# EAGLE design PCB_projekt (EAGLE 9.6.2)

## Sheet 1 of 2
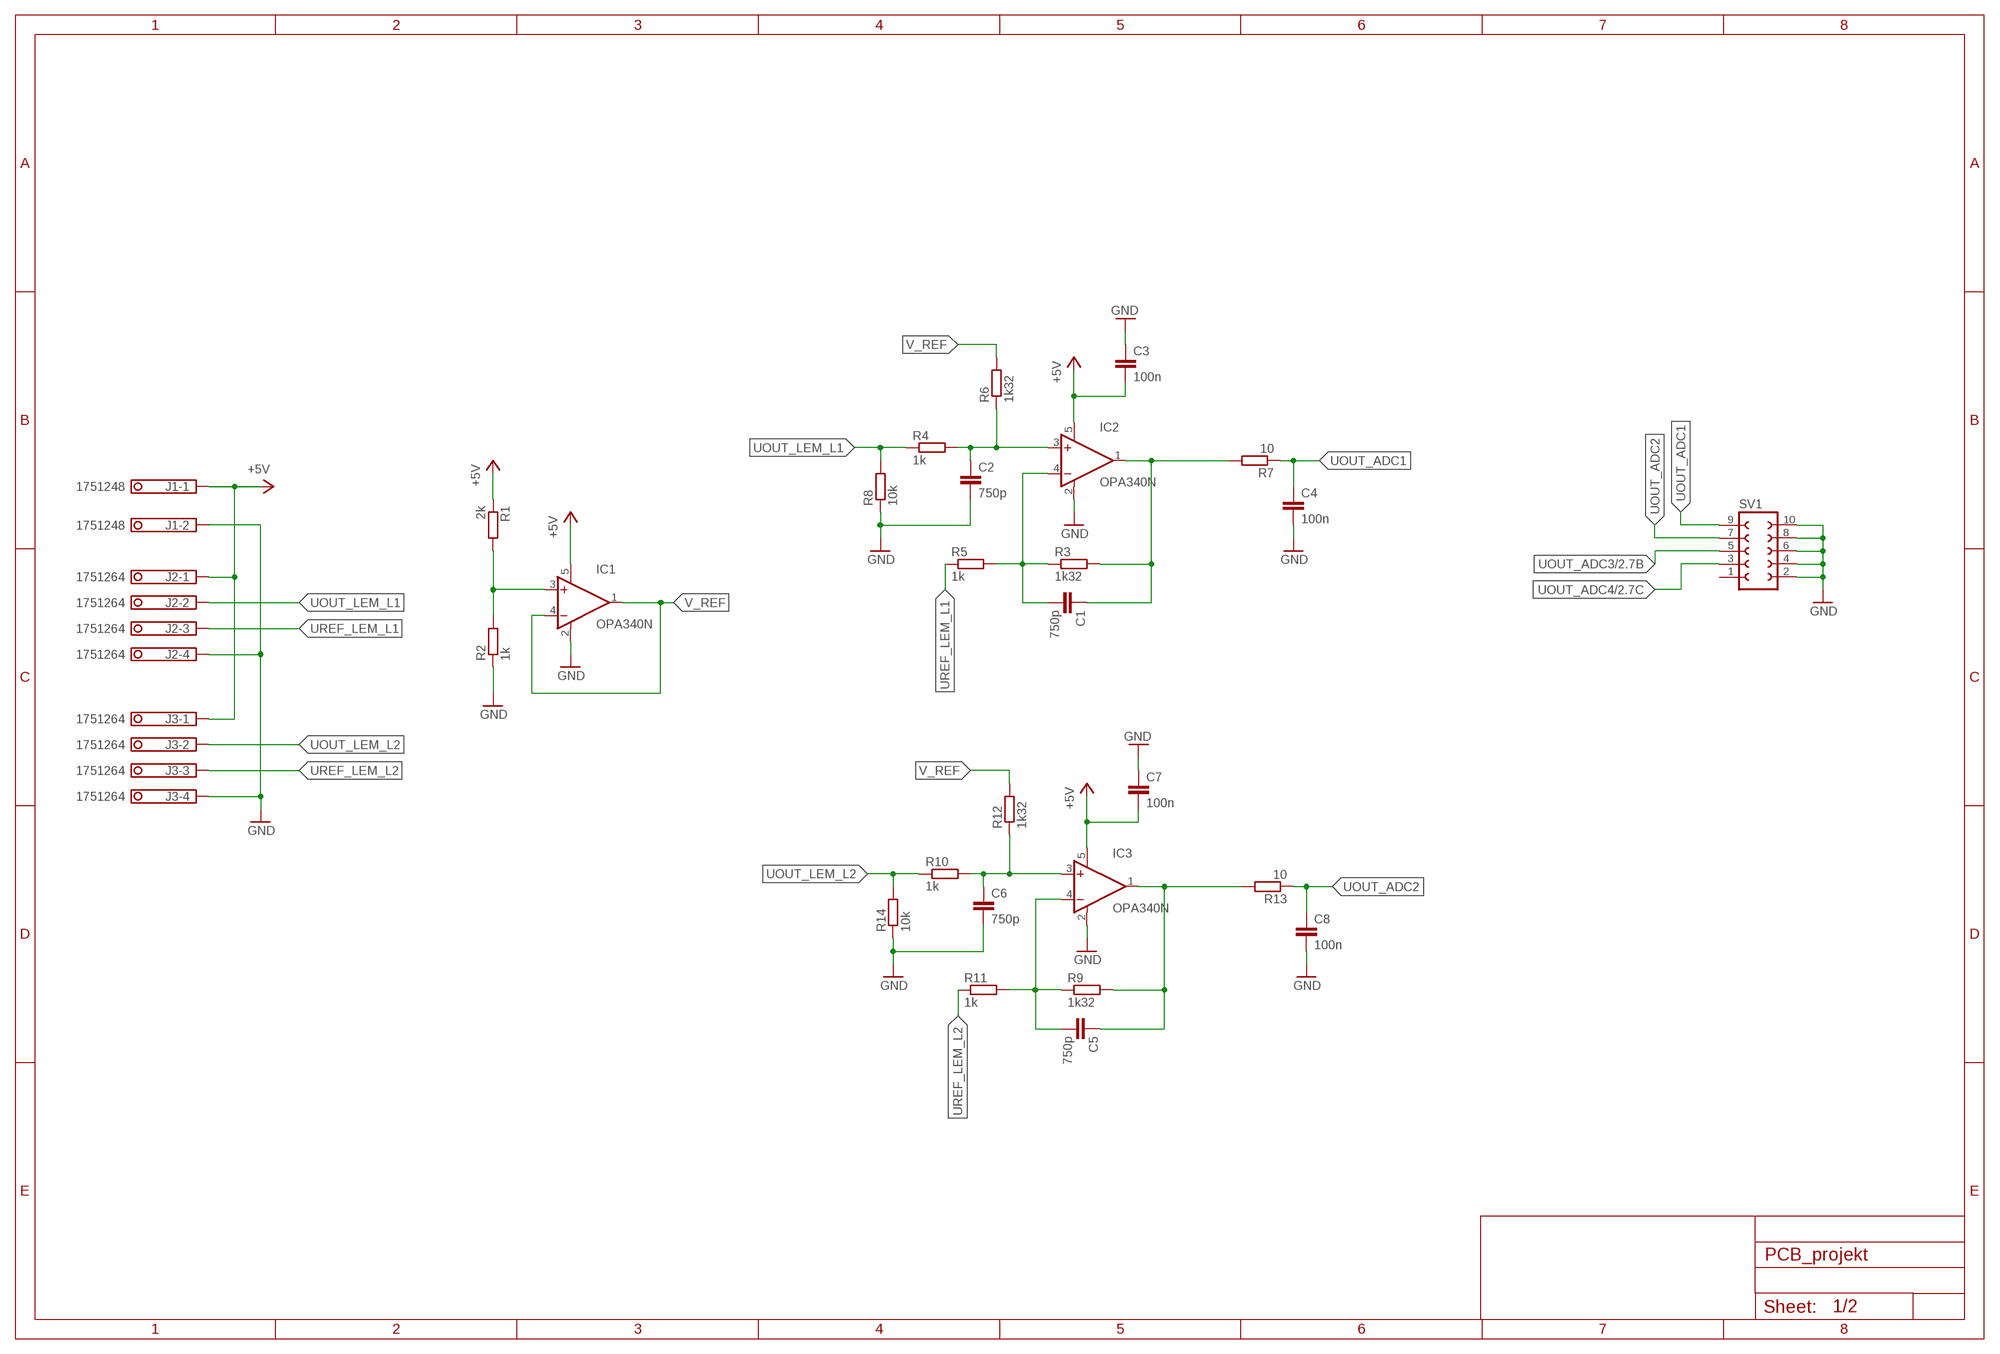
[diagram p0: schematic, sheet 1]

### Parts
C1  750p  C-EUC0603  [C0603]
C2  750p  C-EUC0603  [C0603]
C3  100n  C-EUC0603  [C0603]
C4  100n  C-EUC0603  [C0603]
C5  750p  C-EUC0603  [C0603]
C6  750p  C-EUC0603  [C0603]
C7  100n  C-EUC0603  [C0603]
C8  100n  C-EUC0603  [C0603]
IC1  OPA340N  [SOT23-5]
IC2  OPA340N  [SOT23-5]
IC3  OPA340N  [SOT23-5]
J1  1751248  [1751248]
J2  1751264  [1751264]
J3  1751264  [1751264]
R1  2k  R-EU_R1206  [R1206]
R2  1k  R-EU_R1206  [R1206]
R3  1k32  R-EU_R1206  [R1206]
R4  1k  R-EU_R1206  [R1206]
R5  1k  R-EU_R1206  [R1206]
R6  1k32  R-EU_R1206  [R1206]
R7  10  R-EU_R1206  [R1206]
R8  10k  R-EU_R1206  [R1206]
R9  1k32  R-EU_R1206  [R1206]
R10  1k  R-EU_R1206  [R1206]
R11  1k  R-EU_R1206  [R1206]
R12  1k32  R-EU_R1206  [R1206]
R13  10  R-EU_R1206  [R1206]
R14  10k  R-EU_R1206  [R1206]
SV1  FE05-2  [FE05-2]

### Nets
+5V: C3.2 C7.2 IC1.5(V+) IC2.5(V+) IC3.5(V+) J1.1 J2.1 J3.1 R1.1 ; also sheet 2
GND: C2.2 C3.1 C4.2 C6.2 C7.1 C8.2 IC1.2(V-) IC2.2(V-) IC3.2(V-) J1.2 J2.4 J3.4 R2.1 R8.1 R14.1 SV1.2 SV1.4 SV1.6 SV1.8 SV1.10 ; also sheet 2
N$1: C1.2 IC2.4(-IN) R3.1 R5.2
N$2: C1.1 IC2.1(OUT) R3.2 R7.2
N$4: IC1.3(+IN) R1.2 R2.2
N$5: C2.1 IC2.3(+IN) R4.2 R6.1
N$9: C5.2 IC3.4(-IN) R9.1 R11.2
N$10: C5.1 IC3.1(OUT) R9.2 R13.2
N$11: C6.1 IC3.3(+IN) R10.2 R12.1
UOUT_ADC1: C4.1 R7.1 SV1.9
UOUT_ADC2: C8.1 R13.1 SV1.7
UOUT_ADC3: SV1.5 ; also sheet 2
UOUT_ADC4: SV1.3 ; also sheet 2
UOUT_LEM_L1: J2.2 R4.1 R8.2
UOUT_LEM_L2: J3.2 R10.1 R14.2
UREF_LEM_L1: J2.3 R5.1
UREF_LEM_L2: J3.3 R11.1
V_REF: IC1.1(OUT) IC1.4(-IN) R6.2 R12.2
Unconnected: SV1.1

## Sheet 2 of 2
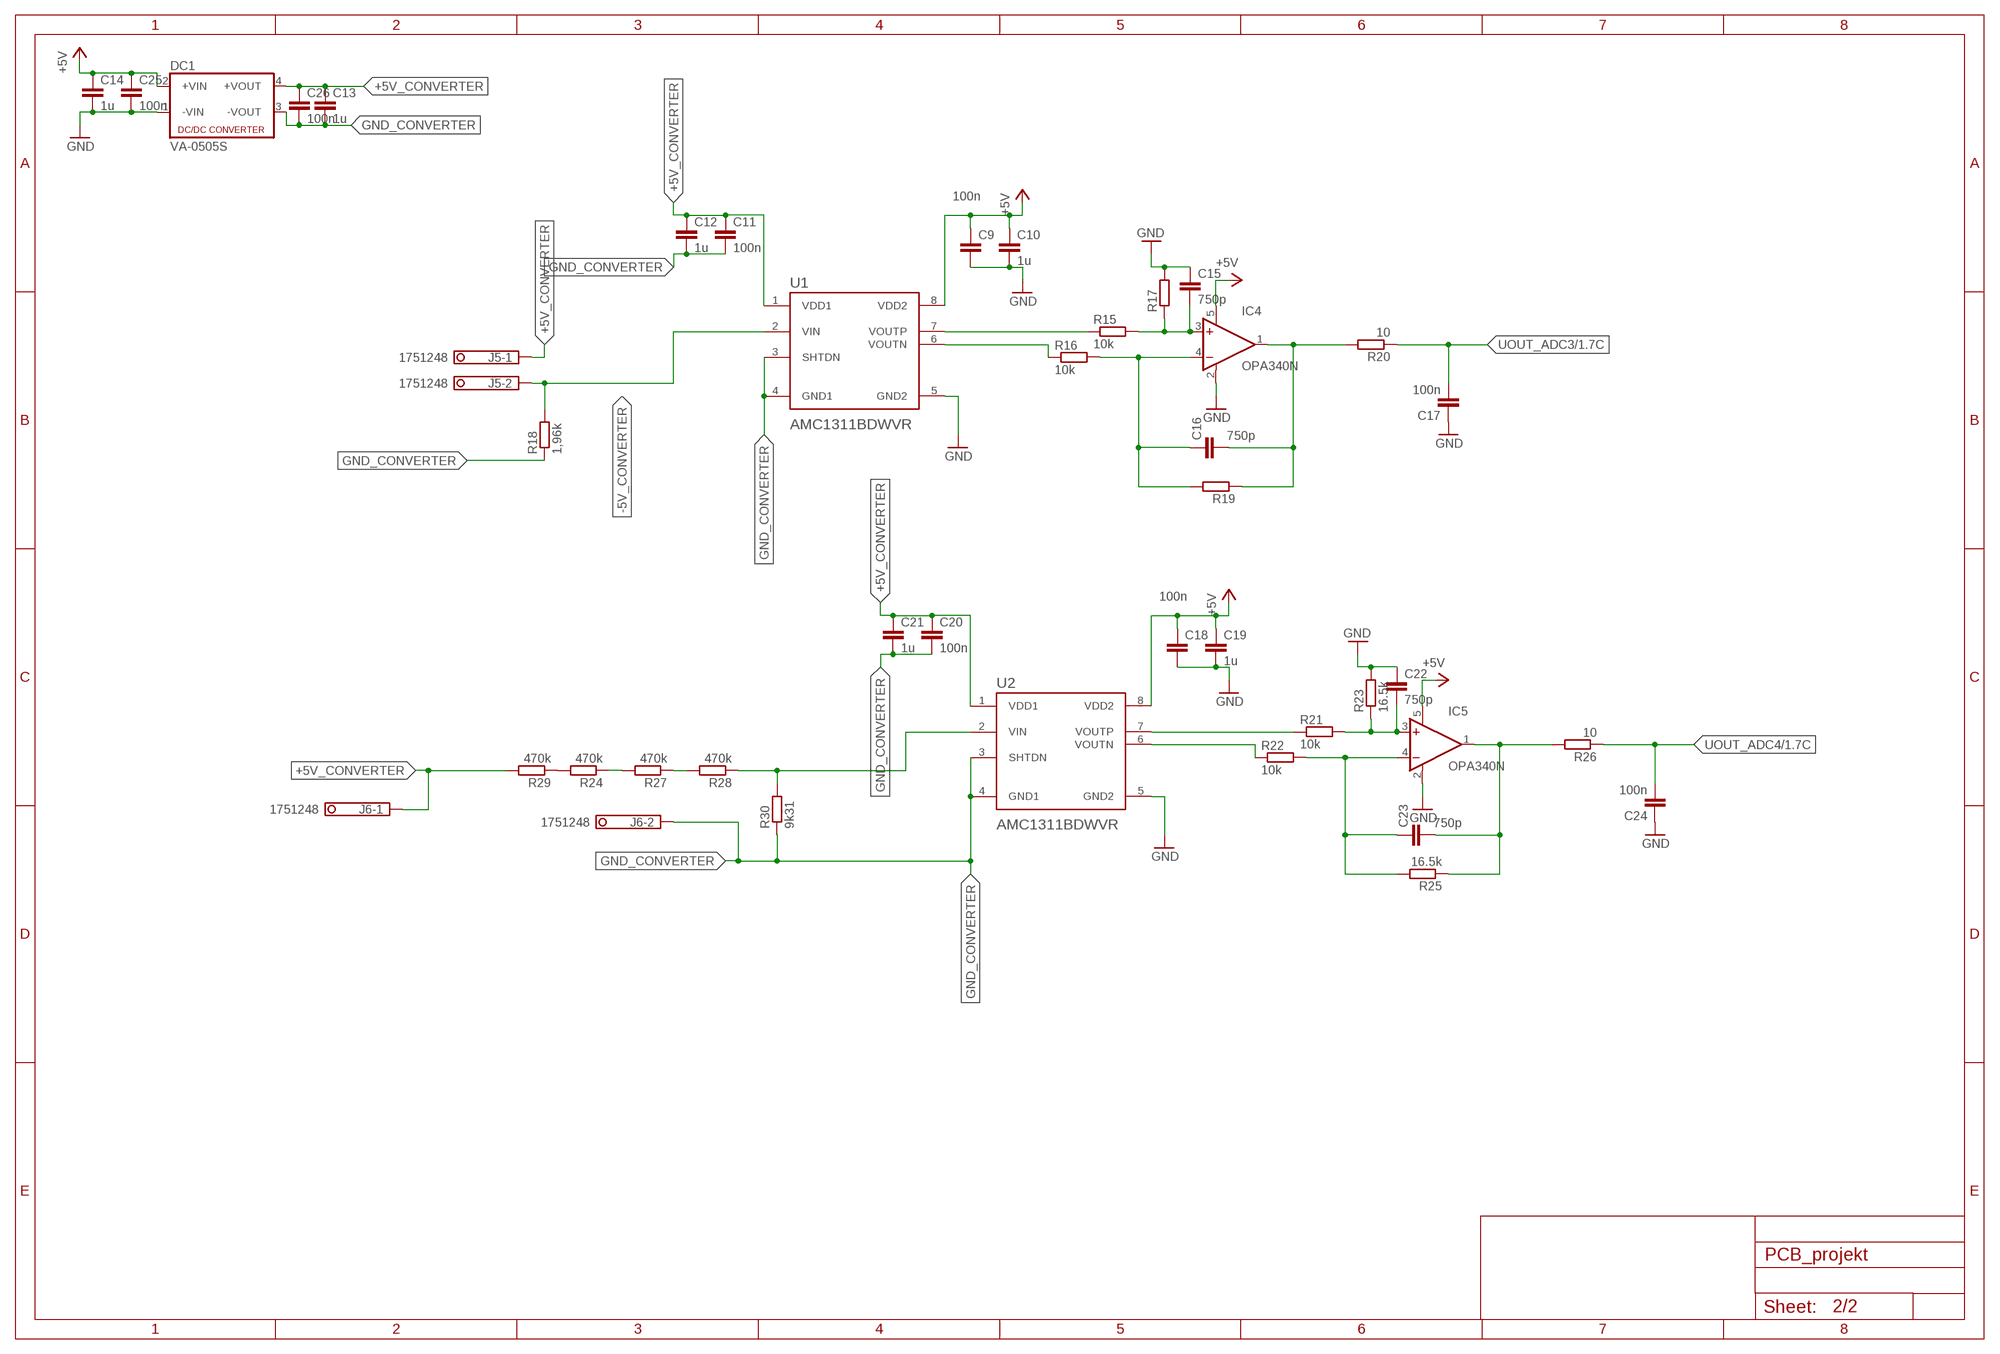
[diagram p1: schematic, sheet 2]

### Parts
C9  100n  C-EUC0603  [C0603]
C10  1u  C-EUC0603  [C0603]
C11  100n  C-EUC0603  [C0603]
C12  1u  C-EUC0603  [C0603]
C13  1u  C-EUC0603  [C0603]
C14  1u  C-EUC0603  [C0603]
C15  750p  C-EUC0603  [C0603]
C16  750p  C-EUC0603  [C0603]
C17  100n  C-EUC0603  [C0603]
C18  100n  C-EUC0603  [C0603]
C19  1u  C-EUC0603  [C0603]
C20  100n  C-EUC0603  [C0603]
C21  1u  C-EUC0603  [C0603]
C22  750p  C-EUC0603  [C0603]
C23  750p  C-EUC0603  [C0603]
C24  100n  C-EUC0603  [C0603]
C25  100n  C-EUC0603  [C0603]
C26  100n  C-EUC0603  [C0603]
DC1  VA-0505S  [4SIL]
IC4  OPA340N  [SOT23-5]
IC5  OPA340N  [SOT23-5]
J5  1751248  [1751248]
J6  1751248  [1751248]
R15  10k  R-EU_R1206  [R1206]
R16  10k  R-EU_R1206  [R1206]
R17  R-EU_R1206  [R1206]
R18  1,96k  R-EU_R1206  [R1206]
R19  R-EU_R1206  [R1206]
R20  10  R-EU_R1206  [R1206]
R21  10k  R-EU_R1206  [R1206]
R22  10k  R-EU_R1206  [R1206]
R23  16.5k  R-EU_R1206  [R1206]
R24  470k  R-EU_R1206  [R1206]
R25  16.5k  R-EU_R1206  [R1206]
R26  10  R-EU_R1206  [R1206]
R27  470k  R-EU_R1206  [R1206]
R28  470k  R-EU_R1206  [R1206]
R29  470k  R-EU_R1206  [R1206]
R30  9k31  R-EU_R1206  [R1206]
U1  AMC1311BDWVR  [SOIC127P1150X280-8N]
U2  AMC1311BDWVR  [SOIC127P1150X280-8N]

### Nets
+5V: C9.1 C10.1 C14.1 C18.1 C19.1 C25.1 DC1.2(+VIN) IC4.5(V+) IC5.5(V+) U1.8(VDD2) U2.8(VDD2) ; also sheet 1
+5V_CONVERTER: C11.1 C12.1 C13.1 C20.1 C21.1 C26.1 DC1.4(+VOUT) J5.1 J6.1 R29.2 U1.1(VDD1) U2.1(VDD1)
-5V_CONVERTER: J5.2 R18.2 U1.2(VIN)
GND: C9.2 C10.2 C14.2 C15.1 C17.1 C18.2 C19.2 C22.1 C24.1 C25.2 DC1.1(-VIN) IC4.2(V-) IC5.2(V-) R17.2 R23.2 U1.5(GND2) U2.5(GND2) ; also sheet 1
GND_CONVERTER: C11.2 C12.2 C13.2 C20.2 C21.2 C26.2 DC1.3(-VOUT) J6.2 R18.1 R30.1 U1.3(SHTDN) U1.4(GND1) U2.3(SHTDN) U2.4(GND1)
N$15: R15.1 U1.7(VOUTP)
N$16: R16.1 U1.6(VOUTN)
N$17: C16.2 IC4.1(OUT) R19.1 R20.2
N$18: C16.1 IC4.4(-IN) R16.2 R19.2
N$19: C15.2 IC4.3(+IN) R15.2 R17.1
N$22: R24.2 R29.1
N$25: R21.1 U2.7(VOUTP)
N$26: R22.1 U2.6(VOUTN)
N$27: C23.2 IC5.1(OUT) R25.1 R26.2
N$28: C23.1 IC5.4(-IN) R22.2 R25.2
N$29: C22.2 IC5.3(+IN) R21.2 R23.1
N$33: R24.1 R27.2
N$34: R27.1 R28.2
N$35: R28.1 R30.2 U2.2(VIN)
UOUT_ADC3: C17.2 R20.1 ; also sheet 1
UOUT_ADC4: C24.2 R26.1 ; also sheet 1

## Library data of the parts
C1-C26 = rcl:C-EU: CAPACITOR, European symbol; SPICEPREFIX: C
DC1 = dc-dc-converter:VA-*?: DC DC Converter Single Output, 1 Watt Motien Technology Co.,Ltd. Source: Data sheet; OC_FARNELL: unknown; OC_NEWARK: unknown
IC1-IC5 = burr-brown:OPA340: Rail-to-Rail Operational Amplifiers Single-Supply, MicroAmplifier(TM) Series; MPN: OPA340NA/3KG4; OC_FARNELL: 1234805; OC_NEWARK: 13M5177
J1 J5 J6 = con-phoenix-350:1751248: MKDS 1/ 2-3,5 Printklemme; OC_FARNELL: unknown; OC_NEWARK: unknown
J2 J3 = con-phoenix-350:1751264: MKDS 1/ 4-3,5 Printklemme Nennstrom: 10 A Bemessungsspannung: 160 V Raster: 3,5 mm Polzahl: 4 Montageart: Löten Anschlussart: Schraubanschluss Anschlussrichtung vom Leiter zur Platine: 0° Source: http://eshop.phoenixcontact.com .. 1751264.pdf; MPN: 1751264; OC_FARNELL: unknown; OC_NEWARK: 10R0934
R1-R30 = rcl:R-EU_: RESISTOR, European symbol; SPICEPREFIX: R
SV1 = con-lsta:FE05-2: FEMALE HEADER; OC_FARNELL: unknown; OC_NEWARK: unknown
U1 U2 = AMC1311BDWVR:AMC1311BDWVR: Check availability; AVAILABILITY: In Stock; CHECK_PRICES: https://www.snapeda.com/parts/AMC1311BDWVR/Texas+Instruments/view-part/?ref=eda; DESCRIPTION: 2-V input, precision voltage sensing reinforced isolated amplifier; MF: Texas Instruments; MP: AMC1311BDWVR; PACKAGE: SOIC-8 Texas Instruments; PRICE: None; PURCHASE-URL: https://www.snapeda.com/api/url_track_click_mouser/?unipart_id=3594462&manufacturer=Texas Instruments&part_name=AMC1311BDWVR&search_term=None; SNAPEDA_LINK: https://www.snapeda.com/parts/AMC1311BDWVR/Texas+Instruments/view-part/?ref=snap

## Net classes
0 default: width 0.3 mm, drill 0.3 mm

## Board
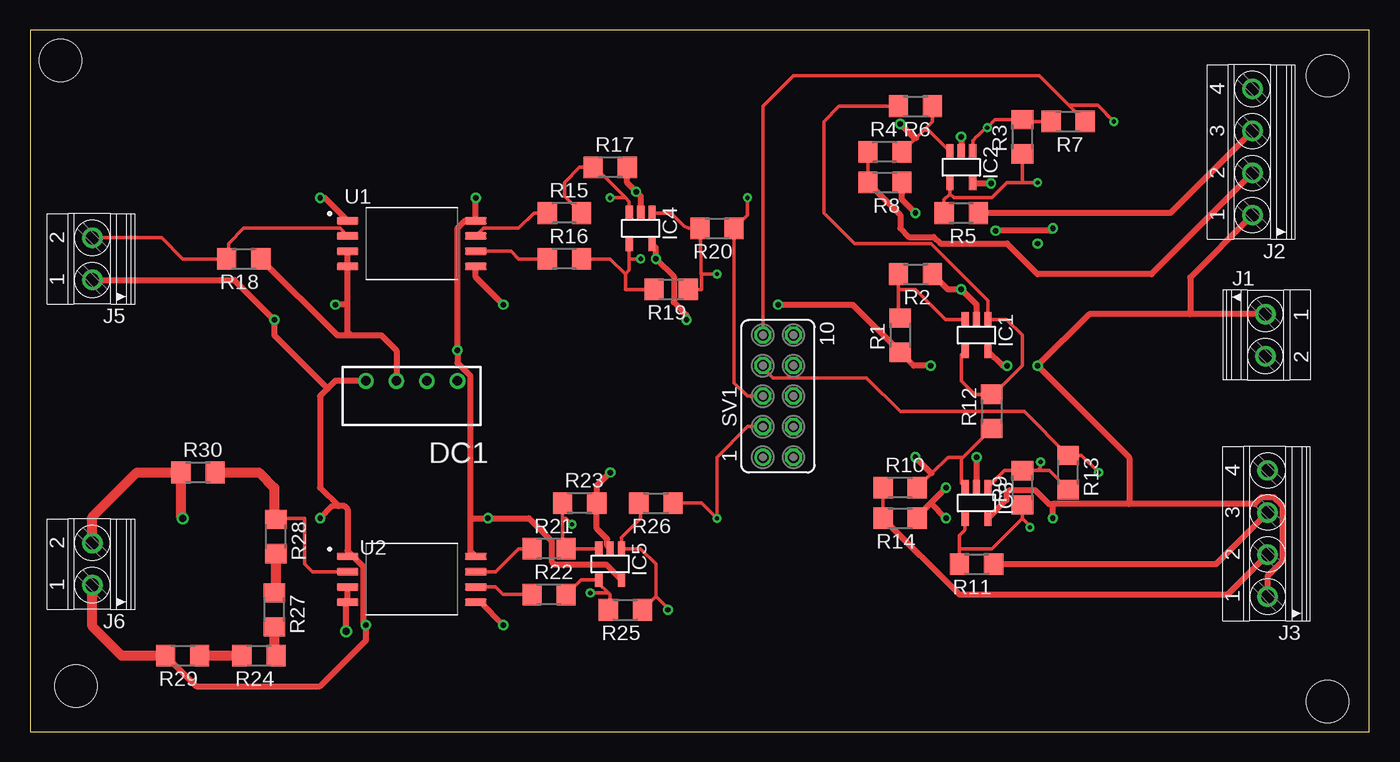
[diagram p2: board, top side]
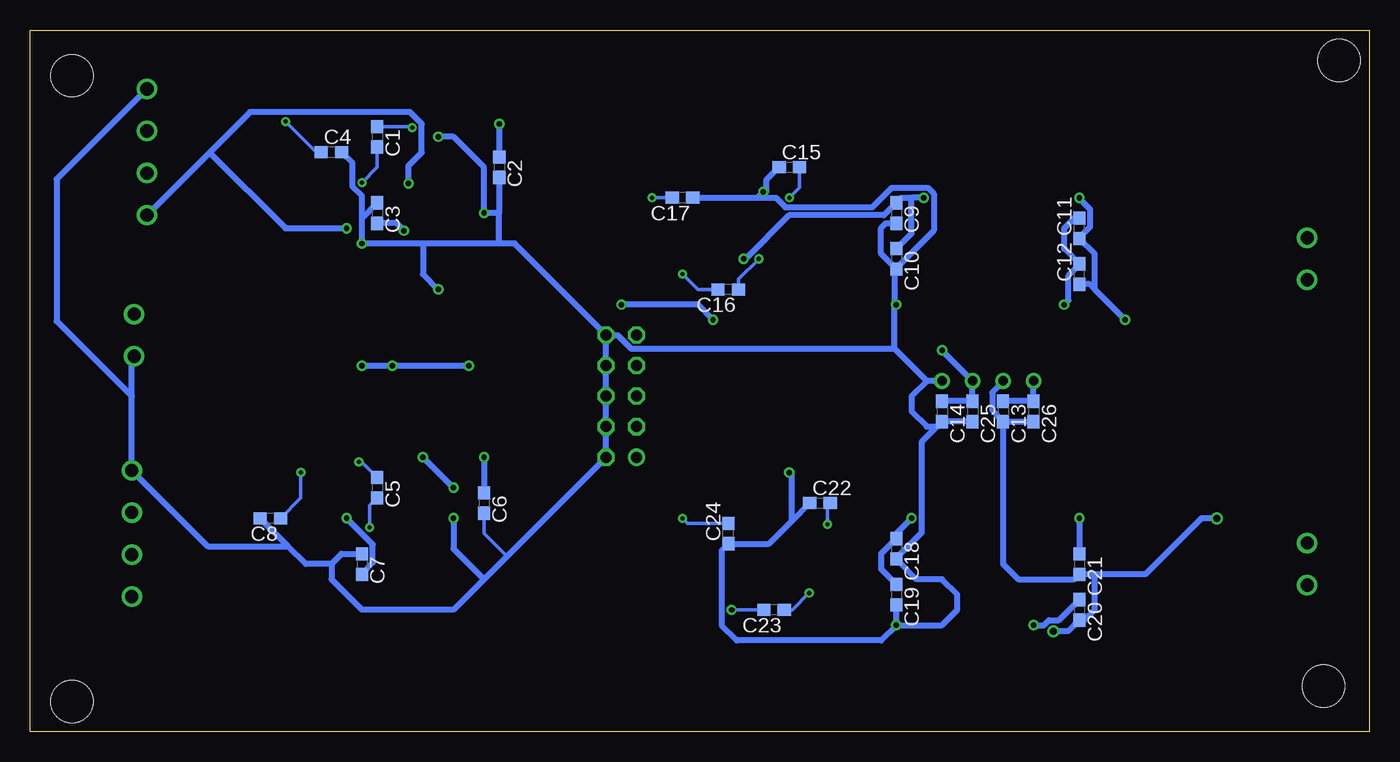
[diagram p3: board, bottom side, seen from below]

Size 111.43 x 58.41 mm. Coordinates in mm from the lower left corner, seen from the top.
Outline: 0,0 111.43,0 111.43,58.41 0,58.41 0,0
Copper layers (1*16): Top 0.035mm / dielectric 1.5mm / Bottom 0.035mm
Design rules "default": minimum track width 6mil, minimum drill 0.35mm, track to track 6mil, track to pad 6mil, pad to pad 6mil, via to via 6mil, smd to smd 6mil, copper to edge 40mil, drill to drill 6mil, minimum pad ring 10mil, minimum via ring 8mil, stop-mask expansion 4mil, vias tented up to drill 0mil, thermal gap 10mil
Holes 3.5 mm at 2.54,55.88 3.81,3.81 107.95,2.54 107.95,54.61

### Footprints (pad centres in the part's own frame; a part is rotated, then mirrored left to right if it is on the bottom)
C0603 = smd 1.1 x 1: 1 -0.85,0; 2 0.85,0
4SIL = drill 0.8: 1 -3.81,0; 2 -1.27,0; 3 1.27,0; 4 3.81,0
SOT23-5 = smd 0.6 x 1.2: 1 -0.95,-1.306; 2 0,-1.306; 3 0.95,-1.306; 4 0.95,1.306; 5 -0.95,1.306
1751248 = drill 1.1 pad 1.7: 1 -1.75,-0.1; 2 1.75,-0.1
1751264 = drill 1.1 pad 1.7: 1 -5.25,-0.1; 2 -1.75,-0.1; 3 1.75,-0.1; 4 5.25,-0.1
R1206 = smd 1.6 x 1.803: 1 -1.422,0; 2 1.422,0
FE05-2 = drill 0.914: 1 -5.08,1.27 | drill 0.914 octagon: 2 -5.08,-1.27; 3 -2.54,1.27; 4 -2.54,-1.27; 5 0,1.27; 6 0,-1.27; 7 2.54,1.27; 8 2.54,-1.27; 9 5.08,1.27; 10 5.08,-1.27
SOIC127P1150X280-8N = smd 1.8 x 0.6: 1 -5.33,1.905; 2 -5.33,0.635; 3 -5.33,-0.635; 4 -5.33,-1.905; 5 5.33,-1.905; 6 5.33,-0.635; 7 5.33,0.635; 8 5.33,1.905

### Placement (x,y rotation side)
C1  82.55,49.53 270 bottom
C2  72.39,46.99 270 bottom
C3  82.55,43.18 270 bottom
C4  86.36,48.26 0 bottom
C5  82.55,20.32 270 bottom
C6  73.66,19.05 270 bottom
C7  83.82,13.97 270 bottom
C8  91.44,17.78 180 bottom
C9  39.37,43.18 270 bottom
C10  39.37,39.37 270 bottom
C11  24.13,41.91 90 bottom
C12  24.13,38.1 90 bottom
C13  30.48,26.67 270 bottom
C14  35.56,26.67 270 bottom
C15  48.26,46.99 0 bottom
C16  53.34,36.83 180 bottom
C17  57.15,44.45 180 bottom
C18  39.37,15.24 270 bottom
C19  39.37,11.43 270 bottom
C20  24.13,10.16 270 bottom
C21  24.13,13.97 270 bottom
C22  45.72,19.05 0 bottom
C23  49.53,10.16 180 bottom
C24  53.34,16.51 90 bottom
C25  33.02,26.67 270 bottom
C26  27.94,26.67 270 bottom
DC1  31.75,29.21 180 top
IC1  78.74,33.02 180 top
IC2  77.47,46.99 180 top
IC3  78.74,19.05 180 top
IC4  50.8,41.91 180 top
IC5  48.26,13.97 180 top
J1  102.87,33.02 270 top
J2  101.6,48.26 90 top
J3  102.87,16.51 90 top
J5  5.08,39.37 90 top
J6  5.08,13.97 90 top
R1  72.39,33.02 90 top
R2  73.66,38.1 180 top
R3  82.55,49.53 90 top
R4  71.12,48.26 0 top
R5  77.47,43.18 180 top
R6  73.66,52.07 180 top
R7  86.36,50.8 180 top
R8  71.12,45.72 180 top
R9  82.55,20.32 90 top
R10  72.39,20.32 0 top
R11  78.74,13.97 180 top
R12  80.01,26.67 90 top
R13  86.36,21.59 270 top
R14  72.39,17.78 180 top
R15  44.45,43.18 0 top
R16  44.45,39.37 0 top
R17  48.26,46.99 0 top
R18  17.78,39.37 180 top
R19  53.34,36.83 180 top
R20  57.15,41.91 180 top
R21  43.18,15.24 0 top
R22  43.18,11.43 0 top
R23  45.72,19.05 0 top
R24  19.05,6.35 180 top
R25  49.53,10.16 180 top
R26  52.07,19.05 180 top
R27  20.32,10.16 270 top
R28  20.45,16.26 270 top
R29  12.7,6.35 180 top
R30  13.97,21.59 0 top
SV1  62.23,27.94 90 top
U1  31.75,40.64 0 top
U2  31.75,12.7 0 top

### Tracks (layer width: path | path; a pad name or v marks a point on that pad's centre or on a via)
+5V  (via drill 0.45)
  Top 0.508: U2.8 36.62,15.07 36.62,17.78 | 36.62,17.78 36.62,29.65 35.56,30.71 v35.56,31.75 35.56,41.91 36.2,42.55 U1.8 v37.08,44.45 | 36.62,17.78 v38.1,17.78 41.49,17.78 43.4,15.88 43.4,14.17 43.63,13.93 47.94,13.93 IC5.5 | IC4.5 52.07,40.28 v52.07,39.37 53.56,37.88 53.56,35.76 54.61,34.71 v54.61,34.29 | v62.23,35.56 68.43,35.56 R1.1 73.51,30.48 v74.93,30.48 | J3.1 102.97,12.98 104.05,14.06 104.23,14.24 104.23,18.78 104.05,18.96 103.49,19.52 102.45,19.52 101.89,18.96 91.44,18.96 | IC3.5 81.24,19.3 81.24,19.87 81.48,20.1 83.62,20.1 84.76,18.96 85.09,18.96 | 91.44,18.96 85.09,18.96 | v85.09,17.78 85.09,18.96 | J1.1 96.52,34.77 | 96.52,34.77 88.11,34.77 v83.82,30.48 91.44,22.86 91.44,18.96 | v81.28,30.48 80.92,30.48 IC1.5 | IC2.5 79.91,45.68 v79.94,45.65 | v85.09,41.91 84.9,41.72 v80.33,41.72 | J2.1 96.52,37.83 96.52,34.77
  Bottom 0.508: C14.1 C25.1 DC1.2 v35.56,31.75 | v38.1,17.78 39.37,16.51 C18.1 40.64,14.82 40.64,13.55 C19.1 | 38.1,44.45 38.95,44.45 C9.1 40.41,42.99 48.29,42.99 51.91,39.37 v52.07,39.37 | v37.08,44.45 38.1,44.45 | C10.1 38.1,41.49 38.1,44.45 | v54.61,34.29 55.88,35.56 v62.23,35.56 | C7.2 83.82,13.19 82.91,14.1 82.91,15.6 v85.09,17.78 | v83.82,30.48 v81.28,30.48 v74.93,30.48 | 96.48,48.22 93.12,51.58 79.81,51.58 78.84,50.62 78.84,48.22 79.94,47.12 v79.94,45.65 | 96.48,48.22 J2.1 | 96.48,48.22 90.17,41.91 v85.09,41.91 | v80.33,41.72 80.95,42.33 C3.2
+5V_CONVERTER  (via drill 0.45)
  Top 0.508: DC1.4 25.4,29.21 24.77,28.57 | 24.77,28.57 24.13,27.94 24.13,20.32 25.65,18.8 | 25.65,18.8 26.16,18.8 26.42,18.54 26.42,15.07 | 26.42,15.07 U2.1 | 25.65,18.8 25.15,18.8 v24.13,17.78 | 24.77,28.57 20.32,33.02 v20.32,34.29 16.99,37.62 J5.1 | v24.13,44.45 24.52,44.45 U1.1 | 26.42,15.07 27.73,13.76 27.73,9.1 v27.94,8.89 27.94,7.62 24.13,3.81 13.82,3.81 R29.2
  Top 0.813: R29.2 7.62,6.35 5.18,8.79 J6.1
  Bottom 0.508: v24.13,17.78 C21.1 | DC1.4 C26.1 C13.1 | v20.32,34.29 22.86,36.83 | 22.86,36.83 23.28,37.25 C12.1 | 22.86,36.83 22.86,39.79 C11.1 24.13,41.14 23.22,42.04 23.22,43.48 24.13,44.38 v24.13,44.45 | v27.94,8.89 27.07,8.89 26.67,9.29 25.85,9.29 C20.1
-5V_CONVERTER
  Top 0.3: J5.2 10.95,41.12 12.7,39.37 R18.2 16.43,39.45 16.51,39.52 16.51,40.64 17.78,41.91 25.79,41.91 U1.2
GND  (via drill 0.45)
  Top 0.508: v39.37,8.89 37.47,10.79 U2.5 | IC5.2 48.02,15.52 48.02,16.04 47.14,16.92 R23.2 47.14,20.47 v48.26,21.59 | v39.37,35.56 37.08,37.85 U1.5 | IC4.2 50.8,44.58 v50.42,44.96 49.68,45.69 R17.2 | v78.74,22.86 IC3.2 | R2.1 76.35,36.83 v77.47,36.83 78.74,35.56 IC1.2 | v73.66,43.18 72.54,44.3 R8.1 | v77.47,49.53 IC2.2 | 74.93,19.05 73.81,17.93 R14.1 | 74.93,19.05 v76.2,17.78 | 74.93,19.05 v76.2,20.32
  Bottom 0.3: C6.2 73.45,17.99 73.66,17.78 73.66,16.51 71.75,14.61
  Bottom 0.508: DC1.1 36.83,29.21 | 36.83,29.21 38.1,27.94 38.1,26.67 36.83,25.4 35.98,25.4 C14.2 | C25.2 C14.2 | 39.16,14.18 C18.2 39.16,14.6 | 39.16,14.18 37.68,12.7 35.56,12.7 34.29,11.43 34.29,10.16 35.56,8.89 v39.37,8.89 | v39.37,8.89 C19.2 | 48.05,17.57 49.96,15.66 C24.1 53.9,15.1 53.9,8.89 52.63,7.62 40.64,7.62 v39.37,8.89 | 48.05,17.57 C22.1 | SV1.10 SV1.8 SV1.6 SV1.4 SV1.2 71.75,14.61 73.66,12.7 | SV1.10 62.54,33.02 61.42,31.9 39.52,31.9 | 36.83,29.21 39.52,31.9 | 39.52,31.9 39.52,35.41 | 39.52,35.41 v39.37,35.56 | C10.2 39.52,38.37 39.52,35.41 | C10.2 40.64,39.79 40.64,41.91 40.22,42.33 C9.2 | C17.1 50.93,44.45 | 50.93,44.45 v50.42,44.96 50.19,44.96 50.19,45.91 C15.1 | 50.93,44.45 49.37,44.45 48.59,43.66 41.36,43.66 39.74,45.28 36.73,45.28 36.24,44.8 36.24,41.72 39.37,38.59 C10.2 | SV1.10 71.12,40.64 72.39,40.64 | 72.39,40.64 78.74,40.64 | 78.74,40.64 v83.82,40.64 83.82,42.76 | 83.82,42.76 C3.1 | 83.82,42.76 83.82,44.61 84.61,45.39 84.61,47.35 C4.2 | 72.39,40.64 72.39,43.18 | C2.2 72.39,43.18 | 73.66,12.7 76.2,10.16 83.82,10.16 86.36,12.7 86.36,13.97 | 86.36,13.97 85.51,14.82 C7.1 | 86.36,13.97 88.48,13.97 89.96,15.45 | 89.96,15.45 C8.2 | 89.96,15.45 96.66,15.45 J3.4 102.97,27.94 | 102.97,27.94 102.97,31.07 J1.2 | J2.4 109.22,45.99 109.22,34.19 102.97,27.94 | 78.74,40.64 78.74,38.1 v77.47,36.83 | 72.39,43.18 v73.66,43.18 73.66,46.99 76.2,49.53 v77.47,49.53 | v76.2,17.78 76.2,15.24 73.66,12.7 | 48.05,17.57 48.05,21.38 v48.26,21.59 | 39.16,14.6 39.16,14.18 | C14.2 37.27,24.11 37.27,16.57 39.16,14.68 39.16,14.6 | v76.2,20.32 v78.74,22.86
GND_CONVERTER  (via drill 0.45, 0.6)
  Top 0.508: v26.29,8.38 26.29,10.66 U2.4 U2.3 | R18.1 25.55,33.02 26.67,33.02 | 26.67,33.02 29.21,33.02 30.48,31.75 DC1.3 | 26.67,33.02 26.42,33.27 26.42,35.56 | 26.42,35.56 U1.4 U1.3 | 26.42,35.56 v25.4,35.56
  Top 0.813: J6.2 5.18,17.88 8.89,21.59 R30.1 12.55,17.93 v12.7,17.78
  Bottom 0.508: v12.7,17.78 13.97,17.78 18.63,13.12 22.86,13.12 | 22.86,13.12 C21.2 24.55,12.7 29.21,12.7 30.48,13.97 C13.2 | 22.86,13.12 22.86,10.16 23.71,9.31 C20.2 25.06,8.38 v26.29,8.38 | DC1.3 30.48,29.14 31.39,28.24 31.39,26.8 30.48,25.89 C13.2 | C13.2 C26.2 | v25.4,35.56 25.04,35.92 25.04,37.97 24.13,38.88 C12.2 25.4,40.22 25.4,41.91 24.55,42.76 C11.2
N$1  (via drill 0.35)
  Top 0.3: IC2.4 76.52,44.77 | R5.2 76.05,44.3 76.52,44.77 | 76.52,44.77 76.84,44.45 80.01,44.45 81.28,45.72 82.55,45.72 | 82.55,45.72 R3.1 | 82.55,45.72 v83.82,45.72
  Bottom 0.3: C1.2 82.55,46.99 v83.82,45.72
N$2  (via drill 0.35)
  Top 0.3: IC2.1 78.42,49.21 78.74,49.53 78.89,49.68 79.5,50.29 v79.63,50.29 80.29,50.95 R3.2 82.7,50.8 R7.2
  Bottom 0.3: C1.1 79.72,50.38 v79.63,50.29
N$4
  Top 0.3: IC1.3 76.16,34.33 73.66,36.83 72.24,36.83 | R1.2 72.24,34.59 72.24,36.83 | R2.2 72.24,36.83
N$5  (via drill 0.45)
  Top 0.3: R4.2 73.74,49.45 74.37,50.09 | 74.37,50.09 75.08,50.8 R6.1 | IC2.3 74.73,50.09 74.37,50.09
  Top 0.508: 73.74,49.45 73.52,49.45 v72.39,50.59
  Bottom 0.508: v72.39,50.59 C2.1
N$9  (via drill 0.35)
  Top 0.3: IC3.4 77.79,16.83 77.32,16.36 77.32,15.24 | 77.32,15.24 R11.2 | R9.1 82.55,17.78 | 77.32,15.24 80.01,15.24 82.55,17.78 | 82.55,17.78 83.19,17.14 v83.19,17.02
  Bottom 0.3: v83.19,17.02 83.19,18.83 C5.2
N$10  (via drill 0.35)
  Top 0.3: IC3.1 81.08,21.74 R9.2 83.82,21.74 | R13.2 84.79,21.74 83.82,21.74 | 83.82,21.74 84.07,22 v84.07,22.48
  Bottom 0.3: v84.07,22.48 83.86,22.48 C5.1
N$11  (via drill 0.45)
  Top 0.3: R10.2 75.01,21.51 76.35,22.86 77.47,22.86 | IC3.3 77.47,20.68 77.47,22.86 | 77.47,22.86 77.62,22.86 R12.1
  Top 0.508: 75.01,21.51 v73.66,22.86
  Bottom 0.508: v73.66,22.86 C6.1
N$15
  Top 0.3: U1.7 37.72,41.91 40.64,41.91 41.91,43.18 R15.1
N$16
  Top 0.3: U1.6 40.01,40 40.64,39.37 R16.1
N$17  (via drill 0.35)
  Top 0.3: R19.1 55.88,36.83 55.88,38.1 | IC4.1 51.79,43.18 53.34,43.18 54.41,42.11 54.77,41.91 R20.2 55.79,41.85 55.83,38.1 55.88,38.1 | 55.88,38.1 v57.15,38.1
  Bottom 0.3: v57.15,38.1 55.88,36.83 C16.2
N$18  (via drill 0.35)
  Top 0.3: R16.2 48.26,39.37 49.53,38.1 | 49.53,38.1 49.53,36.83 R19.2 | IC4.4 49.85,39.37 | 49.85,39.37 49.85,38.42 49.53,38.1 | 49.85,39.37 v50.8,39.37
  Bottom 0.3: v50.8,39.37 52.49,37.68 C16.1
N$19  (via drill 0.35)
  Top 0.3: R15.2 44.45,44.6 44.45,45.72 45.72,46.99 R17.1 46.99,46.99 49.53,44.45 | 49.53,44.45 49.85,44.13 IC4.3 | 49.53,44.45 v48.26,44.45
  Bottom 0.3: v48.26,44.45 47.41,45.3 C15.2
N$22
  Top 0.813: R24.2 R29.1
N$25
  Top 0.3: U2.7 38.73,13.33 40.64,15.24 R21.1
N$26
  Top 0.3: U2.6 38.73,12.07 39.37,11.43 R22.1
N$27  (via drill 0.45)
  Top 0.3: R25.1 52.07,11.28 | 52.07,11.28 52.07,13.97 50.8,15.24 49.25,15.24 IC5.1 49.21,16.19 50.8,17.78 50.8,18.9 R26.2 | 52.07,11.28 53.07,10.28 v53.07,10.16
  Bottom 0.3: v53.07,10.16 C23.2
N$28  (via drill 0.35)
  Top 0.3: R22.2 45.84,12.66 IC5.4 47.31,12.38 48.13,11.56 | R25.2 48.26,10.31 48.26,11.43 48.13,11.56 | v46.61,11.56 48.13,11.56
  Bottom 0.3: v46.61,11.56 48.01,10.16 C23.1
N$29  (via drill 0.35)
  Top 0.3: IC5.3 47.27,15.24 R21.2 44.3,15.54 44.3,17.78 | 44.3,17.78 R23.1 | 44.3,17.78 44.58,17.78 v45.09,17.27
  Bottom 0.3: v45.09,17.27 45.09,18.83 C22.2
N$33
  Top 0.813: R27.2 20.32,6.5 R24.1
N$34
  Top 0.813: R28.2 20.45,11.71 R27.1
N$35
  Top 0.3: U2.2 23.5,13.33 22.86,13.97 22.86,17.78 20.55,17.78 R28.1
  Top 0.813: R30.2 19.05,21.59 20.32,20.32 20.32,17.81 R28.1
UOUT_ADC1  (via drill 0.35)
  Top 0.3: R7.1 86.44,52.15 | 86.44,52.15 83.97,54.61 63.5,54.61 60.96,52.07 SV1.9 | 86.44,52.15 88.82,52.15 v90.17,50.8
  Bottom 0.3: v90.17,50.8 87.63,48.26 C4.1
UOUT_ADC2  (via drill 0.35)
  Top 0.3: SV1.7 60.96,30.32 61.81,29.47 69.59,29.47 72.39,26.67 82.7,26.67 R13.1 87.48,23.01 v88.9,21.59
  Bottom 0.3: v88.9,21.59 88.9,19.47 C8.1
UOUT_ADC3  (via drill 0.35)
  Top 0.3: SV1.5 59.69,27.94 58.57,29.06 R20.1 59.69,43.03 v59.69,44.45
  Bottom 0.3: v59.69,44.45 C17.2
UOUT_ADC4  (via drill 0.35)
  Top 0.3: R26.1 55.88,19.05 v57.15,17.78 57.15,22.86 59.69,25.4 SV1.3
  Bottom 0.3: v57.15,17.78 56.73,17.36 C24.2
UOUT_LEM_L1
  Top 0.3: R4.1 R8.2
  Top 0.508: R8.2 72.39,43.03 72.39,41.91 73.1,41.2 75.16,41.2 75.72,40.64 81.28,40.64 83.82,38.1 93.29,38.1 J2.2
UOUT_LEM_L2
  Top 0.3: R10.1 R14.2
  Top 0.508: R14.2 77.32,11.43 99.64,11.43 J3.2
UREF_LEM_L1
  Top 0.508: J2.3 94.87,43.18 R5.1
UREF_LEM_L2
  Top 0.508: R11.1 98.68,13.97 J3.3
V_REF
  Top 0.3: R6.2 67.31,52.07 66.04,50.8 66.04,43.18 68.58,40.64 74.93,40.64 79.69,35.88 IC1.1 81.24,34.33 82.55,33.02 82.55,30.48 80.28,28.21 80.19,28.27 R12.2 78.59,28.09 77.47,29.21 77.47,31.39 IC1.4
